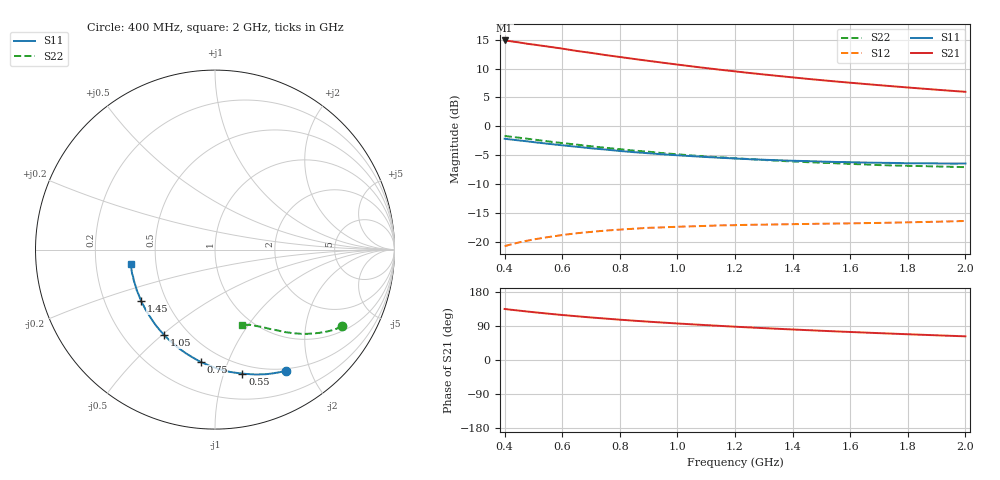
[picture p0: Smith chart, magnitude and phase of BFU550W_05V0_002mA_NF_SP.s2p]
! Filename:  P:\Prog\Test\Noise\ATS_data\Testdata_Net\06 Compressed Noise after Statistics\BFU550W_APM2013_11_D05_05p0V_002mA_NF_CM01_D.sf
! Date/Time: Tue 26/Mar/2013 16:25:21
! BFU550W_APM2013_11_D05_05p0V_1to35mA_NF_CM01_Bias2_R.sf
! Noise Parameter Data File
! BFU550W_APM2013_11_D05_05p0V_1to35mA_NF_CM01
! Date/time: Mon Mar 25 13:26:50 2013
! VAR V_out= 5.000000
! VAR I_out= 1.995000
! VAR V_in= 0.791600
! VAR I_in= 0.020305
! Device data file deembeded for feedlines and parallel
! Original file: \06 Compressed Noise after Statistics\BFU550W_APM2013_11_D05_05p0V_002mA_NF_CM01_R.sf
! Feed-files: PR019V01_070313_Feed1.s2p, PR019V01_070313_Feed2.s2p
! Parallel-file: PR019V01_070313_Par.s2p
# MHz S MA R 50
!  Freq-MHz  S11-mag  S11-arg  S21-mag  S21-arg  S12-mag  S12-arg  S22-mag  S22-arg
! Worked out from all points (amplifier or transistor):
!   37 points, 400 MHz to 2 GHz, reference 50 ohm
!   highest |S21| = 14.8 dB at 400 MHz (marker M1)
!   |S21| within 3 dB of that: start of sweep to 821.3 MHz
!   unconditionally stable (mu >= 1): nowhere
!   at 500 MHz: K = 0.29, MSG = 16.8 dB, |S12| = -19.5 dB
!   at 1.1 GHz: K = 0.60, MSG = 13.6 dB, |S12| = -17.2 dB
!   at 2 GHz: K = 0.97, MSG = 11.2 dB, |S12| = -16.3 dB
!   lowest NFmin = 0.47 dB at 420 MHz
!   S11 on the Smith chart (normalised r, x): 400 MHz: 0.47, -1.64; 550 MHz: 0.42, -1.16; 750 MHz: 0.39, -0.80; 1.05 GHz: 0.37, -0.51; 1.45 GHz: 0.36, -0.28; 2 GHz: 0.36, -0.08
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400  0.7824 -59.8  5.523 134.7  0.09242 57.1  0.8266 -31.2
420  0.7716 -62.3  5.443 132.8  0.09539 56.0  0.8155 -32.3
460  0.7521 -67.2  5.265 129.5  0.1008 53.7  0.7934 -34.4
480  0.7421 -69.5  5.166 127.9  0.1032 52.7  0.782 -35.4
500  0.7319 -72.0  5.093 126.2  0.1056 51.8  0.7709 -36.4
550  0.7081 -77.5  4.893 122.4  0.1106 49.6  0.7432 -38.6
600  0.6867 -83.0  4.697 118.8  0.1153 47.5  0.718 -40.6
650  0.6672 -87.8  4.486 115.5  0.1195 45.8  0.6967 -42.3
700  0.6473 -92.8  4.316 112.2  0.1227 44.2  0.6737 -44.2
750  0.6312 -97.3  4.132 109.3  0.126 42.8  0.6543 -45.6
800  0.6136 -101.7  3.976 106.4  0.1285 41.6  0.6355 -47.1
850  0.599 -106.0  3.823 103.7  0.1308 40.5  0.6181 -48.4
950  0.5736 -113.8  3.547 98.7  0.1343 38.8  0.5871 -50.9
1050  0.5535 -120.9  3.299 94.2  0.1371 37.6  0.561 -53.0
1150  0.5358 -127.8  3.083 89.9  0.1397 36.6  0.5413 -54.9
1200  0.5284 -130.8  2.988 87.9  0.1404 36.4  0.5303 -56.0
1300  0.5153 -136.8  2.809 84.1  0.1418 36.1  0.5131 -57.8
1450  0.502 -145.0  2.577 78.8  0.1437 36.2  0.4914 -60.5
1500  0.4969 -147.6  2.509 77.1  0.1444 36.3  0.4859 -61.3
1600  0.491 -152.7  2.383 74.0  0.1454 36.9  0.4745 -63.1
1750  0.4837 -159.4  2.219 69.4  0.1476 38.2  0.4601 -65.5
2000  0.4777 -170.0  1.99 62.4  0.1525 40.9  0.4449 -70.0
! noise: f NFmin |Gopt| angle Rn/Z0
400  0.4763  0.4687  31.41  0.1764
460  0.5172  0.4697  36.32  0.174
600  0.578  0.4753  45.42  0.1758
800  0.6087  0.4608  61.95  0.1532
1000  0.7046  0.476  76.28  0.1465
1200  0.7453  0.4641  89.67  0.1363
1400  0.7614  0.4825  108.5  0.106
1600  0.7011  0.4795  121.2  0.0885
1800  0.8772  0.4869  134.8  0.0757
2000  0.9276  0.4659  151.5  0.0653
